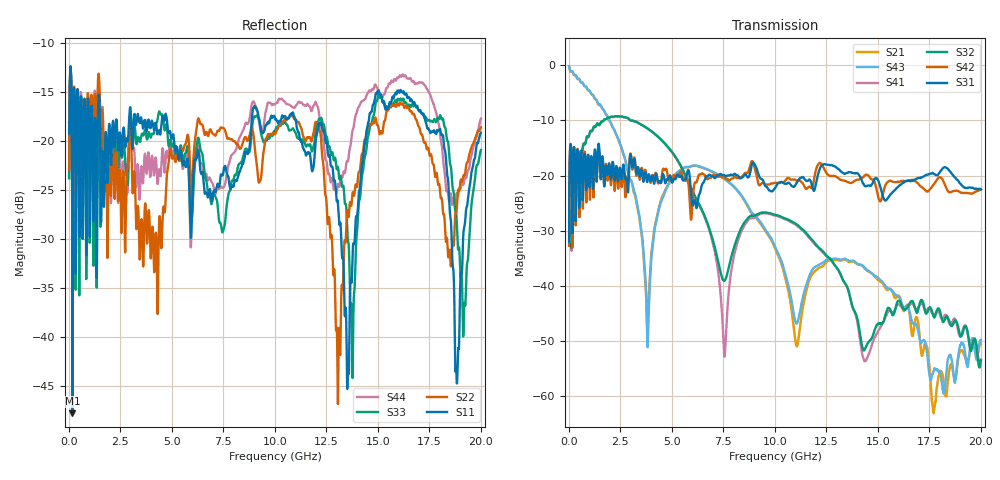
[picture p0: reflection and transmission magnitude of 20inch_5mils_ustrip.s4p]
! FILE: C:\Archive\FR4 ustrip trace\5mils\20inch_5mils_ustrip.s4p
# MHz S DB R 50.00
! FREQ  S11  S12  S13  S14
!  S21  S22  S23  S24
!  S31  S32  S33  S34
!  S41  S42  S43  S44
!  DB  ANG  DB  ANG  DB  ANG  DB  ANG
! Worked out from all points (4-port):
!   2000 points, 10 MHz to 20 GHz, reference 50 ohm
!   strongest paths, dB at 10 MHz, 5.01 GHz, 10.01 GHz, 15.01 GHz, 20 GHz:
!     S31: -32.0, -21.3, -22.2, -20.9, -22.5
!     S42: -32.7, -20.6, -21.3, -23.8, -22.5
!     S32: -28.1, -15.7, -27.1, -46.9, -53.5
!     S41: -30.5, -15.8, -27.3, -48.2, -53.3
!     S43: -0.3, -20.6, -32.9, -38.6, -49.8
!     S21: -0.2, -20.5, -33.2, -38.9, -50.5
!   lowest |S11| = -47.7 dB at 170 MHz (marker M1), VSWR 1.01, Z = 50.4 - j0.147 ohm
!   |S11| at or under -10 dB: start of sweep to end of sweep
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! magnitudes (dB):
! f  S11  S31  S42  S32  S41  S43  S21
! 10 MHz  -18.1  -32.0  -32.7  -28.1  -30.5  -0.3  -0.2
! 170 MHz  -47.7  -30.5  -33.0  -25.9  -25.9  -1.1  -1.1
! 3.83 GHz  -18.3  -20.8  -20.3  -11.5  -11.5  -50.3  -46.2
! 7.55 GHz  -22.6  -19.9  -20.2  -39.1  -52.8  -20.5  -20.7
! 9.53 GHz  -18.5  -21.9  -21.6  -26.7  -26.8  -29.8  -30.0
! 18.84 GHz  -44.7  -20.7  -22.7  -46.7  -47.1  -54.5  -54.8
! 20 GHz  -19.2  -22.5  -22.5  -53.5  -53.3  -49.8  -50.5
